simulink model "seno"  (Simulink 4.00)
settings: Solver=ode45  StartTime=0  StopTime=10  RelTol=1e-3

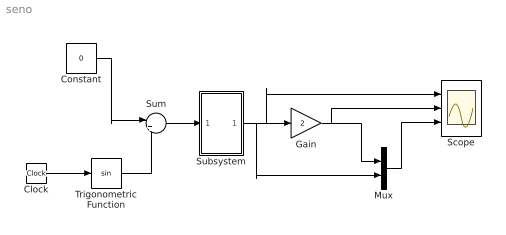
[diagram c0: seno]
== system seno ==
  Clock : Clock
  Constant : Constant  Value=0
  Gain : Gain  Gain=2  Multiplication=Element-wise(K.*u)  SaturateOnIntegerOverflow=on
  Mux : Mux  Inputs=2
  Scope : Scope  NumInputPorts=3
  Subsystem : Subsystem
  Sum : Sum  Inputs=|++  SaturateOnIntegerOverflow=on
  Trigonometric Function : Trigonometry  Operator=sin  OutputSignalType=auto
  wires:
  Constant/1 -> Sum/1
  Trigonometric Function/1 -> Sum/2
  Sum/1 -> Subsystem/1(In1)
  Clock/1 -> Trigonometric Function/1
  Subsystem/1(Out1) -> Mux/2, Gain/1, Scope/1
  Gain/1 -> Mux/1, Scope/2
  Mux/1 -> Scope/3

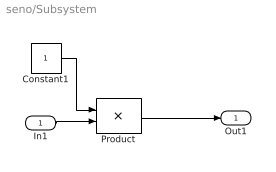
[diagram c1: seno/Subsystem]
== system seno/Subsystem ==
  In1 : Inport  Port=1  LatchInput=off
  Constant1 : Constant  Value=1
  Product : Product  Inputs=2  Multiplication=Element-wise(.*)  SaturateOnIntegerOverflow=on
  Out1 : Outport  Port=1
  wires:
  Constant1/1 -> Product/1
  Product/1 -> Out1/1
  In1/1 -> Product/2
